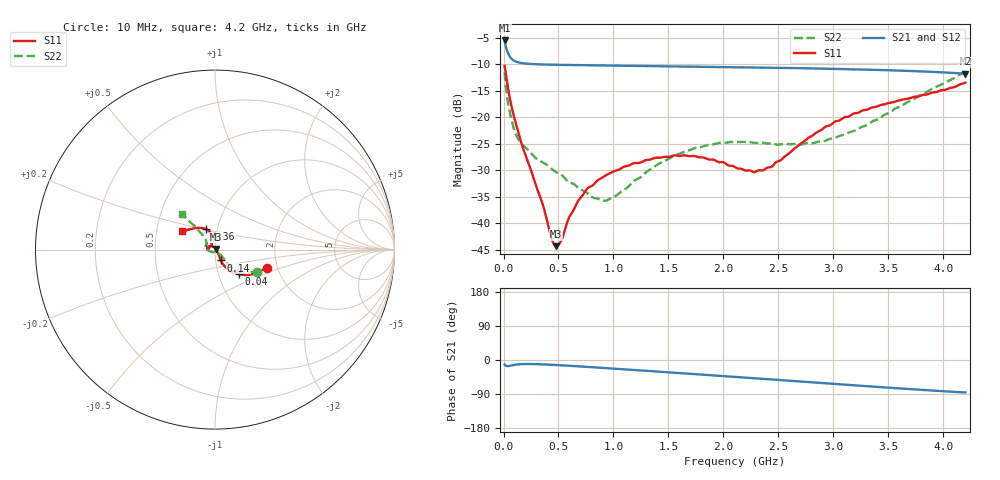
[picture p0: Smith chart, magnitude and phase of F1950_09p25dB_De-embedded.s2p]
! Integrated Device Technology
! Corporate Headquarters
! 6024 Silver Creek Valley Road
! San Jose, CA 95138  USA
! Phone:  1-408-284-8200
! Toll Free:  1-800-223-1366
! Webpage:  http://www.idt.com/
! Timing and RF Division
! 515 Groton Road, Suite 102
! Westford, MA 01886-6024
! Device:  F1950
! Description: 7-bit 0.25 dB Digital Step Attenuator
! Frequency:  150.0 -  4000.00 MHz
! Package:  4x4 mm Thin QFN Plastic Package: 24 pin
! Ports:  2 RF, 12 DC
!  Pin  1  = D0
!  Pin  2  = VDD
!  Pin  3  = Vmode
!  Pin  4  = GND
!  Pin  5  = RF1  =  Port 1
!  Pin  6  = GND
!  Pin  7  = GND
!  Pin  8  = GND
!  Pin  9  = GND
!  Pin 10  = GND
!  Pin 11  = GND
!  Pin 12  = GND
!  Pin 13  = GND
!  Pin 14  = RF2  =  Port 2
!  Pin 15  = GND
!  Pin 16  = LE
!  Pin 17  = CLK
!  Pin 18  = DATE
!  Pin 19  = D6
!  Pin 20  = D5
!  Pin 21  = D4
!  Pin 22  = D3
!  Pin 23  = D2
!  Pin 24  = D1
! State:  37
! Atten State:  9.25 dB
! Voltage:  +5.00 Volts
! Current:  Not Measured mA
! Data:  The device was measured on a the F195X evaluation board which has
!  individual transmission lines to the RF pins.  Data was collected
!  using a calibrated network analyzer.  The evaluation board was
!  de-embedded using a TRL calibration technique.
!  The reference plane is the edge of the package pin.
! Misc:  Board 2019
!  Action Tracker AT0250
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# GHz S dB R 50
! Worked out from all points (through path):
!   420 points, 10 MHz to 4.2 GHz, reference 50 ohm
!   highest |S21| = -5.50 dB at 10 MHz (marker M1); lowest = -11.8 dB at 4.2 GHz (marker M2)
!   group delay of S21, straight-line fit = 53.6 ps
!   lowest |S11| = -44.3 dB at 480 MHz (marker M3), VSWR 1.01, Z = 50.5 + j0.374 ohm
!   |S11| at or under -10 dB: start of sweep to end of sweep
!   |S22| runs from -35.7 to -11.3 dB; largest |S21 - S12| = 0.0004
!   S11 on the Smith chart (normalised r, x): 10 MHz: 1.75, -0.39; 40 MHz: 1.26, -0.36; 140 MHz: 1.06, -0.13; 3.36 GHz: 0.88, +0.20; 4.2 GHz: 0.67, +0.14
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0.01  -10.30 -19.3  -5.50 -12.1  -5.50 -12.1  -11.49 -28.0
0.04  -14.31 -45.5  -7.85 -16.2  -7.85 -16.2  -17.10 -47.1
0.09  -19.43 -59.9  -9.24 -13.3  -9.24 -13.3  -21.85 -47.0
0.14  -23.25 -61.7  -9.66 -11.4  -9.66 -11.3  -24.26 -45.0
0.35  -35.99 -38.9  -10.03 -11.4  -10.02 -11.4  -28.39 -45.3
0.44  -43.04 -1.2  -10.07 -12.6  -10.07 -12.6  -29.73 -46.0
0.48  -44.29 37.4  -10.09 -13.2  -10.09 -13.2  -30.35 -49.0
0.52  -43.42 69.9  -10.10 -13.9  -10.10 -13.9  -30.73 -50.0
0.6  -38.72 102.9  -10.13 -15.3  -10.13 -15.3  -32.24 -55.5
0.71  -34.96 119.2  -10.16 -17.2  -10.16 -17.2  -33.69 -66.6
0.82  -32.67 128.8  -10.19 -19.3  -10.19 -19.3  -35.17 -84.0
0.94  -30.82 138.3  -10.22 -21.6  -10.22 -21.6  -35.66 -109.2
1.41  -27.62 165.8  -10.34 -30.7  -10.34 -30.7  -28.76 -168.9
1.73  -27.28 175.4  -10.42 -37.0  -10.42 -37.0  -25.87 178.1
2.11  -29.44 166.8  -10.53 -44.7  -10.53 -44.8  -24.68 167.8
2.28  -30.34 146.4  -10.58 -48.2  -10.58 -48.2  -24.81 163.2
2.43  -29.39 125.9  -10.63 -51.1  -10.63 -51.2  -24.93 158.9
2.81  -23.42 102.3  -10.77 -59.0  -10.76 -59.0  -24.86 143.9
3.09  -20.07 105.2  -10.89 -64.8  -10.88 -64.8  -23.32 136.3
3.36  -18.10 114.0  -11.03 -70.3  -11.03 -70.3  -20.70 131.6
3.51  -17.26 119.3  -11.12 -73.2  -11.11 -73.3  -19.12 130.5
4.2  -13.45 151.3  -11.77 -85.6  -11.76 -85.7  -11.35 133.4
